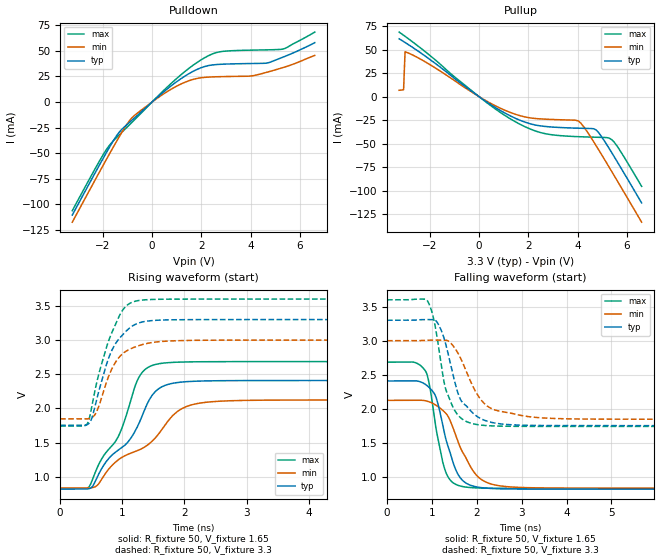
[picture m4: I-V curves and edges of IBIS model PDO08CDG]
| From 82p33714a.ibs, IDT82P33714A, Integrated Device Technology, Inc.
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[Model]   PDO08CDG
Model_type   Output
Polarity   Non-Inverting
|   typ   min   max
C_comp   70.2000fF   57.9000fF   75.6000fF
Vmeas = 1.65V
Rref = 1M
Cref = 0
Vref = 1.65V
|   typ   min   max
[Voltage range]   3.3V   3.0V   3.6V
[Temperature Range]   25.0000   125.00   -40.0000
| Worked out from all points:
|   slope of the pulldown table from 0 to 0.495 V, typ, clamps not added: 47.7 ohm
|   slope of the pullup table from 0 to 0.495 V, typ, clamps not added: 56.1 ohm
|   rising waveform, R_fixture 50, V_fixture 1.65: 20-80 % time 734ps typ, 1.02ns min, 568ps max; typ from 0.82 V to 2.41 V
|   falling waveform, R_fixture 50, V_fixture 1.65: 20-80 % time 384ps typ, 535ps min, 293ps max; typ from 2.41 V to 0.82 V
|   rising waveform, R_fixture 50, V_fixture 3.3: 20-80 % time 355ps typ, 330ps min, 362ps max; typ from 1.75 V to 3.3 V
|   falling waveform, R_fixture 50, V_fixture 3.3: 20-80 % time 439ps typ, 549ps min, 344ps max; typ from 3.3 V to 1.75 V
[Pulldown]
|Voltage   I (typ)   I (min)   I (max)
|Note, modeling breaks down at 250mA and above.  This is well beyond the functional   |
|operating range of the device.  Should this scenario occur, catastrophic failure and   |
|possible damage to the device and/or board is of higher concern than the I-V curve   |
|behavior.  The IBIS checker will flag currents in excess of 10A with warnings.  Lines   |
|with currents in excess of 0.35 A have been commented out.  The points still remain|
|available to the user if the user desires to use them.   |
-3.24V    -110.3mA   -117.3mA   -106.1mA
-1.853V   -49.3mA    -55.96mA   -46.34mA
-1.44V    -32.89mA   -38.28mA   -34.58mA
-1.027V   -22.23mA   -21.93mA   -24.85mA
-716.7mV  -15.6mA    -13.13mA   -17.47mA
316.7mV   6.756mA    5.479mA    7.664mA
1.453V    27.05mA    20.38mA    32.06mA
2.487V    36.26mA    24.5mA     47.26mA
4.037V    37.53mA    25.43mA    50.6mA
4.657V    37.94mA    29.01mA    50.87mA
5.277V    43.41mA    33.33mA    51.47mA
6.6V      57.88mA    45.4mA     68.21mA
[Pullup]
|Voltage   I (typ)   I (min)   I (max)
|Note, modeling breaks down at 250mA and above.  This is well beyond the functional   |
|operating range of the device.  Should this scenario occur, catastrophic failure and   |
|possible damage to the device and/or board is of higher concern than the I-V curve   |
|behavior.  The IBIS checker will flag currents in excess of 10A with warnings.  Lines   |
|with currents in excess of 0.35 A have been commented out.  The points still remain|
|available to the user if the user desires to use them.   |
-3.24V    61.46mA    6.731mA    68.61mA
-3.06V    58.55mA    7.336mA    65.24mA
-3V       57.56mA    47.72mA    64.1mA
-1.957V   38.81mA    33.43mA    43.01mA
110mV     -2.04mA    -1.741mA   -2.287mA
1.35V     -21.52mA   -17.64mA   -24.86mA
2.59V     -31.48mA   -23.87mA   -38.86mA
4.037V    -33.61mA   -26.01mA   -42.63mA
4.76V     -35.58mA   -52.51mA   -43.23mA
5.38V     -59.33mA   -79.38mA   -45.64mA
5.69V     -72.78mA   -93.05mA   -56.02mA
6.6V      -113.1mA   -133.6mA   -95.5mA
[Ramp]
|   typ   min   max
dV/dt_r   0.954/0.734n   0.774/1.018n   1.113/0.569n
dV/dt_f   0.954/0.384n   0.775/0.535n   1.114/0.293n
R_load =   50.0000
[Rising Waveform]
R_fixture = 50
V_fixture = 1.65   |Vcc_typ
V_fixture_min = 1.5 |Vcc_min
V_fixture_max = 1.8 |Vcc_max
C_fixture = 0.0p
| Time   typ   min   max
0s        819.5mV    833.9mV    830.8mV
472.5ps   827mV      834.3mV    861.8mV
664.7ps   1.114V     959.3mV    1.256V
953ps     1.401V     1.259V     1.622V
1.113ns   1.534V     1.337V     2.043V
1.265ns   1.775V     1.39V      2.451V
1.53ns    2.244V     1.566V     2.642V
1.914ns   2.381V     1.972V     2.677V
2.394ns   2.403V     2.094V     2.684V
8ns       2.408V     2.124V     2.685V
[Falling Waveform]
R_fixture = 50
V_fixture = 1.65   |Vcc_typ
V_fixture_min = 1.5 |Vcc_min
V_fixture_max = 1.8 |Vcc_max
C_fixture = 0.0p
| Time   typ   min   max
0s        2.408V     2.124V     2.685V
608.6ps   2.411V     2.124V     2.682V
864.9ps   2.354V     2.117V     2.545V
953ps     2.304V     2.099V     2.321V
1.081ns   2.185V     2.056V     1.752V
1.265ns   1.684V     1.963V     1.158V
1.586ns   1.032V     1.509V     875mV
2.002ns   851.6mV    1.018V     837.5mV
2.49ns    825.6mV    870.5mV    831.9mV
8ns       819.5mV    833.9mV    830.8mV
[Rising Waveform]
R_fixture = 50
V_fixture = 3.3   |Vcc_typ
V_fixture_min = 3.0 |Vcc_min
V_fixture_max = 3.6 |Vcc_max
C_fixture = 0.0p
| Time   typ   min   max
0s        1.752V     1.846V     1.741V
440.4ps   1.765V     1.847V     1.782V
504.5ps   1.845V     1.863V     2.004V
584.6ps   2.121V     1.948V     2.363V
800.8ps   2.786V     2.516V     3.041V
1.009ns   3.08V      2.803V     3.442V
1.209ns   3.23V      2.9V       3.569V
1.53ns    3.288V     2.97V      3.596V
2.09ns    3.299V     2.995V     3.6V
8ns       3.3V       3V         3.6V
[Falling Waveform]
R_fixture = 50
V_fixture = 3.3   |Vcc_typ
V_fixture_min = 3.0 |Vcc_min
V_fixture_max = 3.6 |Vcc_max
C_fixture = 0.0p
| Time   typ   min   max
0s        3.3V       3V         3.6V
896.9ps   3.31V      3.007V     3.589V
1.049ns   3.307V     3.008V     3.29V
1.185ns   3.187V     3.008V     2.748V
1.321ns   2.916V     3.006V     2.26V
1.594ns   2.204V     2.801V     1.897V
1.826ns   1.998V     2.455V     1.797V
2.25ns    1.813V     2.032V     1.752V
3.091ns   1.758V     1.89V      1.741V
8ns       1.752V     1.846V     1.741V
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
